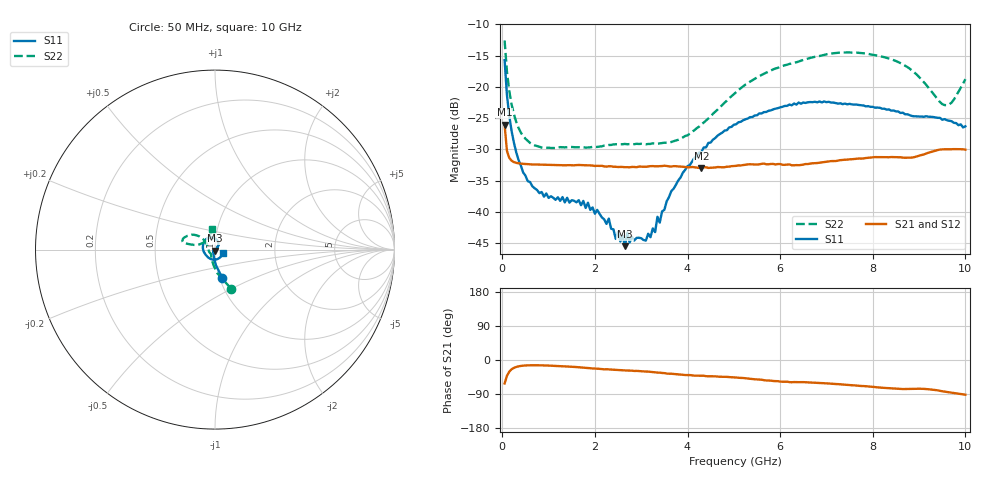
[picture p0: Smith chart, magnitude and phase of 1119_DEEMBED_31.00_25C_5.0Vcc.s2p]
!Hittite Microwave Corp.
!Digital Attenuator/PhaseShifter Rev 1.4.0
!Filename: C:\DATA\DATA\1119_DEEMBED_31.00_25C_5.0Vcc.s2p
!VNA ID: Agilent Technologies,N5224A,MY51441122,A.10.45.03
!Device type:
!2 Port Calibration.
!Temp(C): 25
!Lot Number:
!Serial Number:
!Operator:
!Misc:
!Attenuator:  31.000
# GHZ S DB R 50.0
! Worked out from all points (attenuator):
!   200 points, 50 MHz to 10 GHz, reference 50 ohm
!   highest |S21| = -26.07 dB at 50 MHz (marker M1); lowest = -33.0 dB at 4.3 GHz (marker M2)
!   lowest |S11| = -45.5 dB at 2.65 GHz (marker M3), VSWR 1.01, Z = 49.9 - j0.522 ohm
!   |S11| at or under -10 dB: start of sweep to end of sweep
!   |S22| runs from -29.8 to -12.6 dB; largest |S21 - S12| = 0.00012
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0.05  -15.72 -75.5  -26.07 -61.9  -26.09 -61.9  -12.56 -67.6
0.1  -21.28 -86.8  -30.23 -42.0  -30.21 -42.0  -17.51 -84.0
0.2  -27.03 -97.7  -31.82 -24.5  -31.82 -24.8  -22.78 -100.6
0.55  -35.11 -121.7  -32.37 -14.1  -32.38 -14.1  -28.65 -126.5
0.9  -37.59 -134.9  -32.46 -14.3  -32.47 -14.3  -29.77 -135.9
1.75  -38.27 -141.0  -32.56 -20.2  -32.55 -20.2  -29.68 -140.9
2.3  -41.10 -133.6  -32.71 -24.8  -32.72 -24.9  -29.31 -149.4
2.45  -44.36 -122.5  -32.80 -26.1  -32.82 -26.1  -29.19 -151.0
2.65  -45.52 -99.5  -32.87 -27.4  -32.87 -27.4  -29.14 -154.1
2.7  -43.34 -84.4  -32.86 -27.9  -32.86 -27.9  -29.19 -154.6
2.75  -44.94 -85.0  -32.89 -27.8  -32.89 -27.9  -29.16 -155.6
3.1  -44.63 -32.6  -32.80 -30.5  -32.81 -30.5  -29.20 -164.8
3.3  -43.27 4.1  -32.72 -32.8  -32.71 -32.8  -29.07 -170.7
3.35  -40.81 8.1  -32.72 -33.2  -32.74 -33.2  -29.12 -172.4
3.4  -41.75 14.8  -32.70 -33.4  -32.70 -33.4  -29.06 -173.8
3.65  -36.69 34.2  -32.77 -36.2  -32.77 -36.2  -28.83 177.0
4.3  -30.42 54.1  -32.99 -41.3  -33.01 -41.4  -26.00 150.3
5.05  -25.99 73.4  -32.65 -46.2  -32.66 -46.3  -20.83 138.5
6.7  -22.45 120.9  -32.24 -59.7  -32.26 -59.6  -15.27 153.8
8.35  -23.62 -177.9  -31.27 -74.3  -31.27 -74.4  -15.45 168.1
9.55  -25.16 -79.9  -29.99 -83.5  -30.00 -83.5  -22.91 138.0
10  -26.32 -24.5  -30.06 -91.7  -30.07 -91.7  -18.76 98.1
